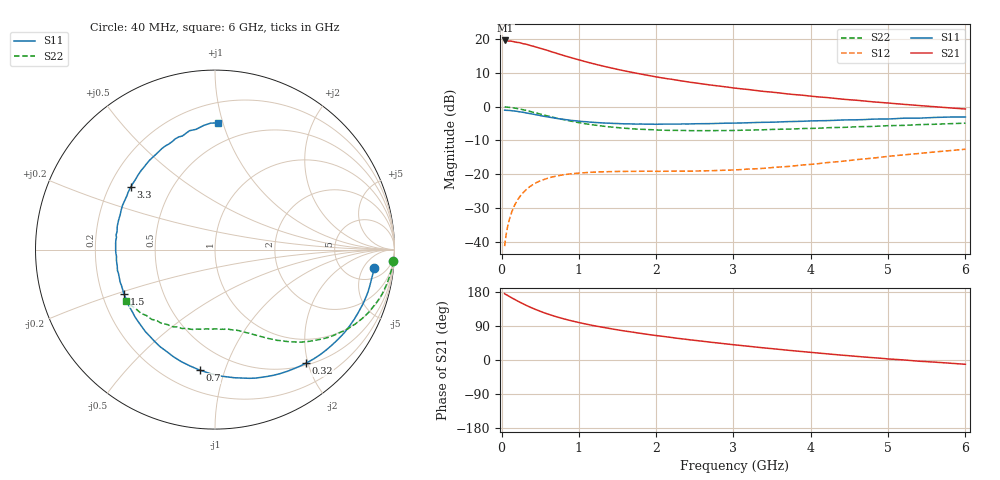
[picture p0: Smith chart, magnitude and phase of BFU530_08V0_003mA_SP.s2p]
! Filename:  P:\Prog\Test\Noise\ATS_data\Testdata_Net\03 Spar\BFU530_APG2013_40_A05_08p0V_003mA_SP_CM01_D.s2p
! Date/Time: Fri 26/Apr/2013 13:03:14
! BFU530_APG2013_40_A05_08p0V_1to25mA_SP_CM01_Bias3_R.s2p
! MDIF S-parameter v. bias file
! BFU530_APG2013_40_A05_08p0V_1to25mA_SP_CM01
! Date/time Wed Apr 24 16:58:28 2013
! VAR V_out= 8.0000
! VAR I_out= 2.9950
! VAR V_in= 0.8041
! VAR I_in= 0.0313
! Device data file deembeded for feedlines and parallel
! Original file: \03 Spar\BFU530_APG2013_40_A05_08p0V_003mA_SP_CM01_R.s2p
! Feed-files: PR047V01_250413_Feed1.s2p, PR047V01_250413_Feed2.s2p
! Parallel-file: PR047V01_250413_Par.s2p
# MHz S MA R 50
!  Freq-MHz  S11-mag  S11-arg  S21-mag  S21-arg  S12-mag  S12-arg  S22-mag  S22-arg
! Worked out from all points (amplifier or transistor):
!   98 points, 40 MHz to 6 GHz, reference 50 ohm
!   highest |S21| = 19.7 dB at 50 MHz (marker M1)
!   |S21| within 3 dB of that: start of sweep to 601.1 MHz
!   unconditionally stable (mu >= 1): 2.599 GHz to 4.573 GHz
!   at 300 MHz: K = 0.14, MSG = 21.8 dB, |S12| = -25.0 dB
!   at 1.6 GHz: K = 0.66, MSG = 14.9 dB, |S12| = -19.2 dB
!   at 6 GHz: K = 0.82, MSG = 6.0 dB, |S12| = -12.6 dB
!   S11 on the Smith chart (normalised r, x): 40 MHz: 9, -9; 320 MHz: 0.53, -1.97; 700 MHz: 0.33, -0.82; 1.5 GHz: 0.29, -0.21; 3.3 GHz: 0.29, +0.31; 6 GHz: 0.34, +0.96
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40  0.8918 -6.7  9.65 175.0  0.008525 86.0  0.994 -3.7
50  0.8904 -8.4  9.665 173.3  0.01055 84.9  0.9934 -4.6
70  0.8867 -11.6  9.562 171.5  0.01475 83.2  0.989 -6.7
120  0.8784 -20.0  9.452 165.5  0.02491 78.3  0.9761 -11.3
220  0.8487 -36.0  9.021 154.3  0.04349 69.4  0.9351 -20.2
320  0.811 -51.2  8.493 144.1  0.05904 61.3  0.8831 -28.1
420  0.7728 -65.0  7.881 135.1  0.07148 54.6  0.8256 -34.8
500  0.742 -75.1  7.401 128.6  0.0795 49.8  0.7819 -39.4
600  0.7065 -86.9  6.849 121.2  0.08721 44.8  0.7301 -44.5
700  0.6766 -97.3  6.294 114.7  0.09304 40.6  0.6847 -48.8
850  0.6405 -111.1  5.577 106.3  0.0996 35.7  0.6273 -54.0
1050  0.6041 -126.9  4.804 96.6  0.1047 30.9  0.5686 -60.0
1200  0.5863 -137.1  4.33 90.4  0.1071 28.2  0.5361 -63.6
1500  0.5649 -154.0  3.598 79.6  0.1096 24.8  0.4916 -69.8
1750  0.554 -166.0  3.144 71.8  0.1102 23.5  0.467 -74.5
2050  0.5525 -177.8  2.72 63.3  0.1102 23.2  0.451 -80.0
2450  0.5578 167.6  2.307 53.0  0.1107 24.3  0.4421 -87.3
3100  0.5754 148.5  1.851 38.2  0.1169 29.3  0.4486 -98.6
3300  0.5853 143.1  1.742 33.9  0.1203 30.9  0.4534 -102.2
4100  0.6205 124.1  1.403 18.3  0.1434 36.0  0.4808 -116.5
5200  0.6774 102.2  1.089 0.2  0.1932 35.9  0.5298 -136.1
6000  0.7066 88.7  0.9277 -11.3  0.2345 31.3  0.5713 -150.1
